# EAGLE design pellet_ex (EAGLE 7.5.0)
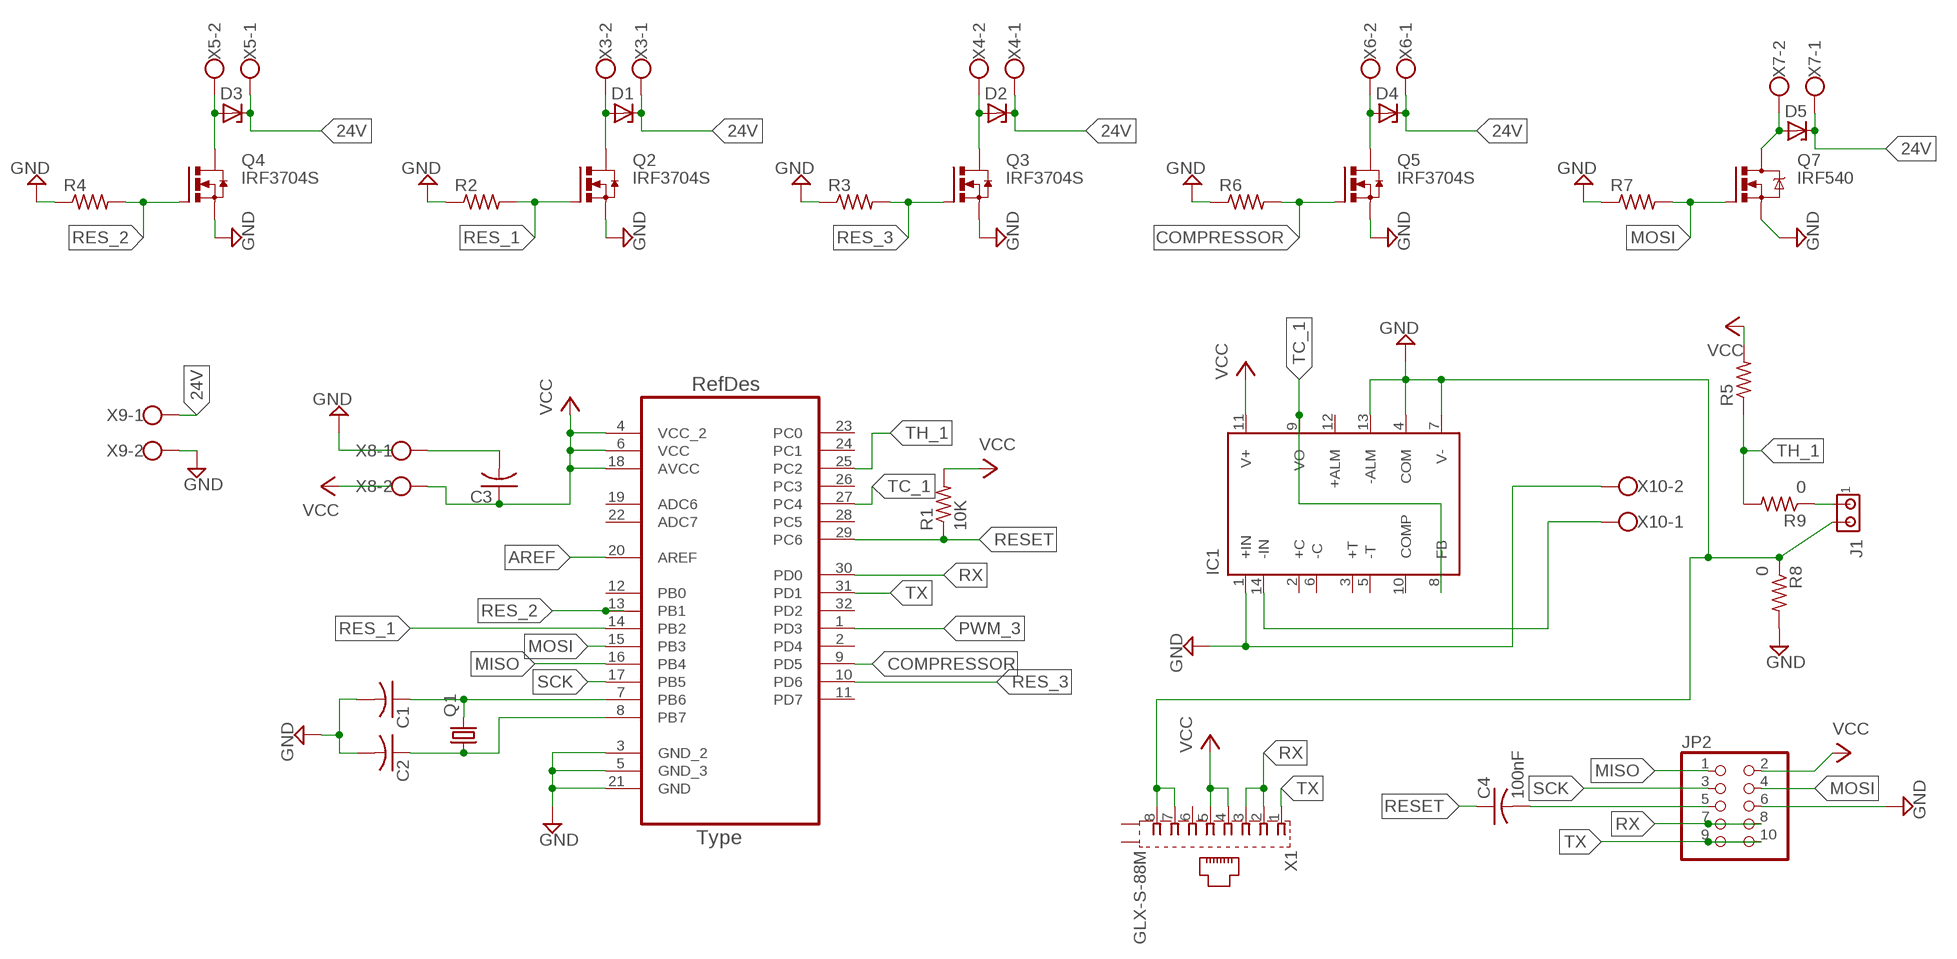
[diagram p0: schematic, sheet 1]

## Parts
C1  C-USC1206K  [C1206K]
C2  C-USC1206K  [C1206K]
C3  C-USC1206K  [C1206K]
C4  100nF  C-USC1206  [C1206]
D1  ZENER_DIODESOD123  [SOD123]
D2  ZENER_DIODESOD123  [SOD123]
D3  ZENER_DIODESOD123  [SOD123]
D4  ZENER_DIODESOD123  [SOD123]
D5  ZENER_DIODESOD123  [SOD123]
IC1  AD594  [DIL14]
J1  MTA02-156  [1X2MTA]
JP2  PINHD-2X5SMT  [2X05_SMT]
Q1  CRYSTALSM49  [SM49]
Q2  IRF3704S  [D2PACK]
Q3  IRF3704S  [D2PACK]
Q4  IRF3704S  [D2PACK]
Q5  IRF3704S  [D2PACK]
Q7  IRF540  [TO220BV]
R1  10K  R-US_M1206  [M1206]
R2  R-US_M1206  [M1206]
R3  R-US_M1206  [M1206]
R4  R-US_M1206  [M1206]
R5  R-US_M1206  [M1206]
R6  R-US_M1206  [M1206]
R7  R-US_M1206  [M1206]
R8  0  R-US_M1206  [M1206]
R9  0  R-US_M1206  [M1206]
U1  ATMEGA328P-AU  [QFP80P900X900X120-32N]
X1  GLX-S-88M  [GLX-S-88M]
X3  W237-102  [W237-102]
X4  W237-102  [W237-102]
X5  W237-102  [W237-102]
X6  W237-102  [W237-102]
X7  W237-102  [W237-102]
X8  W237-102  [W237-102]
X9  W237-102  [W237-102]
X10  W237-102  [W237-102]

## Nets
24V: D1.CATHODE D2.CATHODE D3.CATHODE D4.CATHODE D5.CATHODE X3.1 X4.1 X5.1 X6.1 X7.1 X9.1
AREF: U1.20(AREF)
COMPRESSOR: Q5.1(G) R6.2 U1.9(PD5)
GND: C1.2 C2.2 IC1.1(+IN) IC1.4(COM) IC1.7(V-) IC1.13(-ALM) J1.2 JP2.6 Q2.3(S) Q3.3(S) Q4.3(S) Q5.3(S) Q7.S R2.1 R3.1 R4.1 R6.1 R7.1 R8.1 R8.2 U1.3(GND_2) U1.5(GND_3) U1.21(GND) X1.7 X1.8 X9.2 X10.2
MISO: JP2.1 U1.16(PB4)
MOSI: JP2.4 Q7.G R7.2 U1.15(PB3)
N$1: IC1.14(-IN) X10.1
N$2: C1.1 Q1.2 U1.7(PB6)
N$3: C2.1 Q1.1 U1.8(PB7)
N$4: D1.ANODE Q2.2(D) X3.2
N$5: D2.ANODE Q3.2(D) X4.2
N$6: D3.ANODE Q4.2(D) X5.2
N$7: C4.2 JP2.5
N$8: D4.ANODE Q5.2(D) X6.2
N$9: D5.ANODE Q7.D X7.2
N$10: C3.2 X8.1
N$13: J1.1 R9.1
PWM_3: U1.1(PD3)
RES_1: Q2.1(G) R2.2 U1.14(PB2)
RES_2: Q4.1(G) R4.2 U1.13(PB1)
RES_3: Q3.1(G) R3.2 U1.10(PD6)
RESET: C4.1 R1.1 U1.29(PC6)
RX: JP2.7 JP2.8 U1.30(PD0) X1.2 X1.3
SCK: JP2.3 U1.17(PB5)
TC_1: IC1.8(FB) IC1.9(VO) U1.27(PC4)
TH_1: R5.1 R9.2 U1.25(PC2)
TX: JP2.9 JP2.10 U1.31(PD1) X1.1
VCC: C3.1 IC1.11(V+) JP2.2 R1.2 R5.2 U1.4(VCC_2) U1.6(VCC) U1.18(AVCC) X1.4 X1.5 X8.2
Unconnected: IC1.2(+C) IC1.3(+T) IC1.5(-T) IC1.6(-C) IC1.10(COMP) IC1.12(+ALM) U1.2(PD4) U1.11(PD7) U1.12(PB0) U1.19(ADC6) U1.22(ADC7) U1.23(PC0) U1.24(PC1) U1.26(PC3) U1.28(PC5) U1.32(PD2) X1.6 X1.S1 X1.S2

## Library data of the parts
C1-C4 = adafruit:C-US: CAPACITOR, American symbol
D1-D5 = fab:ZENER_DIODE: zener diode
IC1 = analog-devices:AD594: ANALOG DEVICES; MF: ALTERA CORPORATION; MPN: AD594AQ; OC_FARNELL: 409182; OC_NEWARK: 05F7088
J1 = con-amp:MTA02-156: AMP connector
JP2 = pinhead+:PINHD-2X5: PIN HEADER
Q1 = adafruit:CRYSTAL: CRYSTAL; OC_FARNELL: unknown; OC_NEWARK: unknown
Q2-Q5 = transistor-power:IRF3704: SMPS MOSFET HEXFET® Power MOSFET Source: http://www.irf.com/product-info/datasheets/data/irf3704.pdf
Q7 = transistor-power:IRF540: HEXFET Power MOSFET
R1-R9 = adafruit:R-US_: RESISTOR, American symbol
U1 = ATMEGA328P-AU:ATMEGA328P-AU; DESCRIPTION: 8-bit Microcontroller with In-System Programmable Flash; MPN: ATMEGA328P-AU; OC_FARNELL: 1715486; OC_NEWARK: 14R4631; PACKAGE: TQFP-32; SUPPLIER: Atmel
X1 = con-kycon:GLX-S-88M: Mod. Jack, Right Angle, 8 posiotion, 8 contatcs RJ45 Source: GLX-S-88M.pdf; OC_FARNELL: unknown; OC_NEWARK: unknown
X3-X10 = con-wago-500:W237-102: WAGO SCREW CLAMP; MPN: 237-102; OC_FARNELL: unknown; OC_NEWARK: 70K9898

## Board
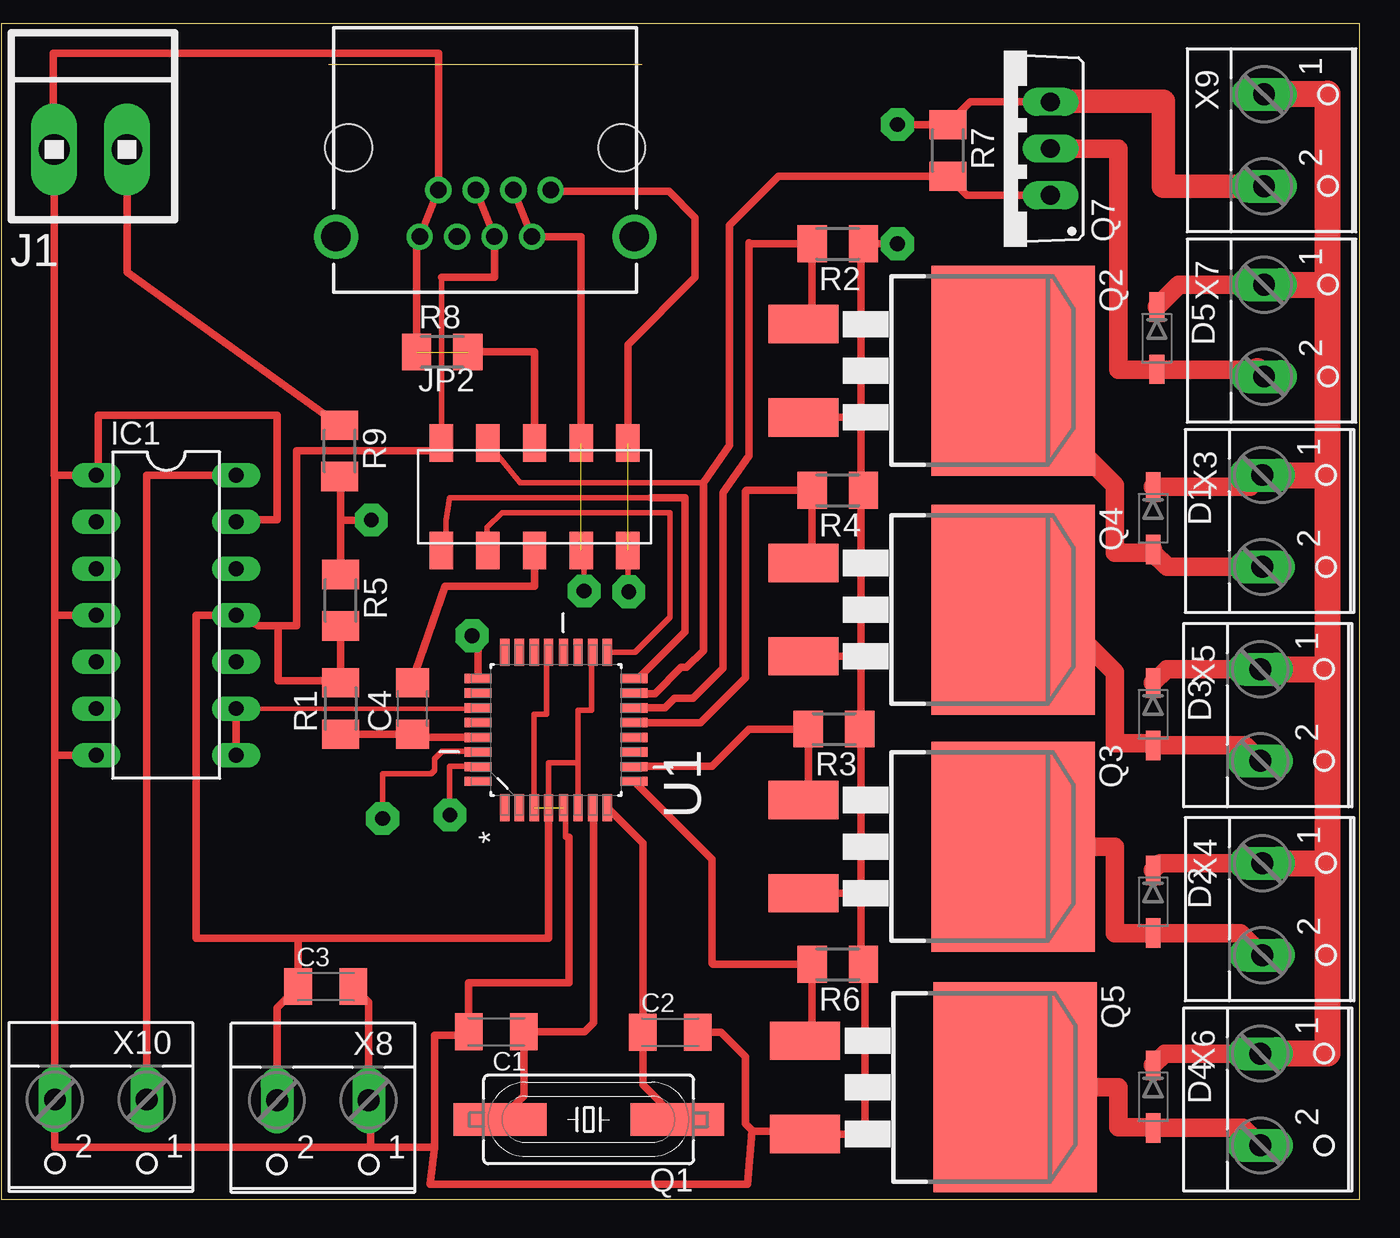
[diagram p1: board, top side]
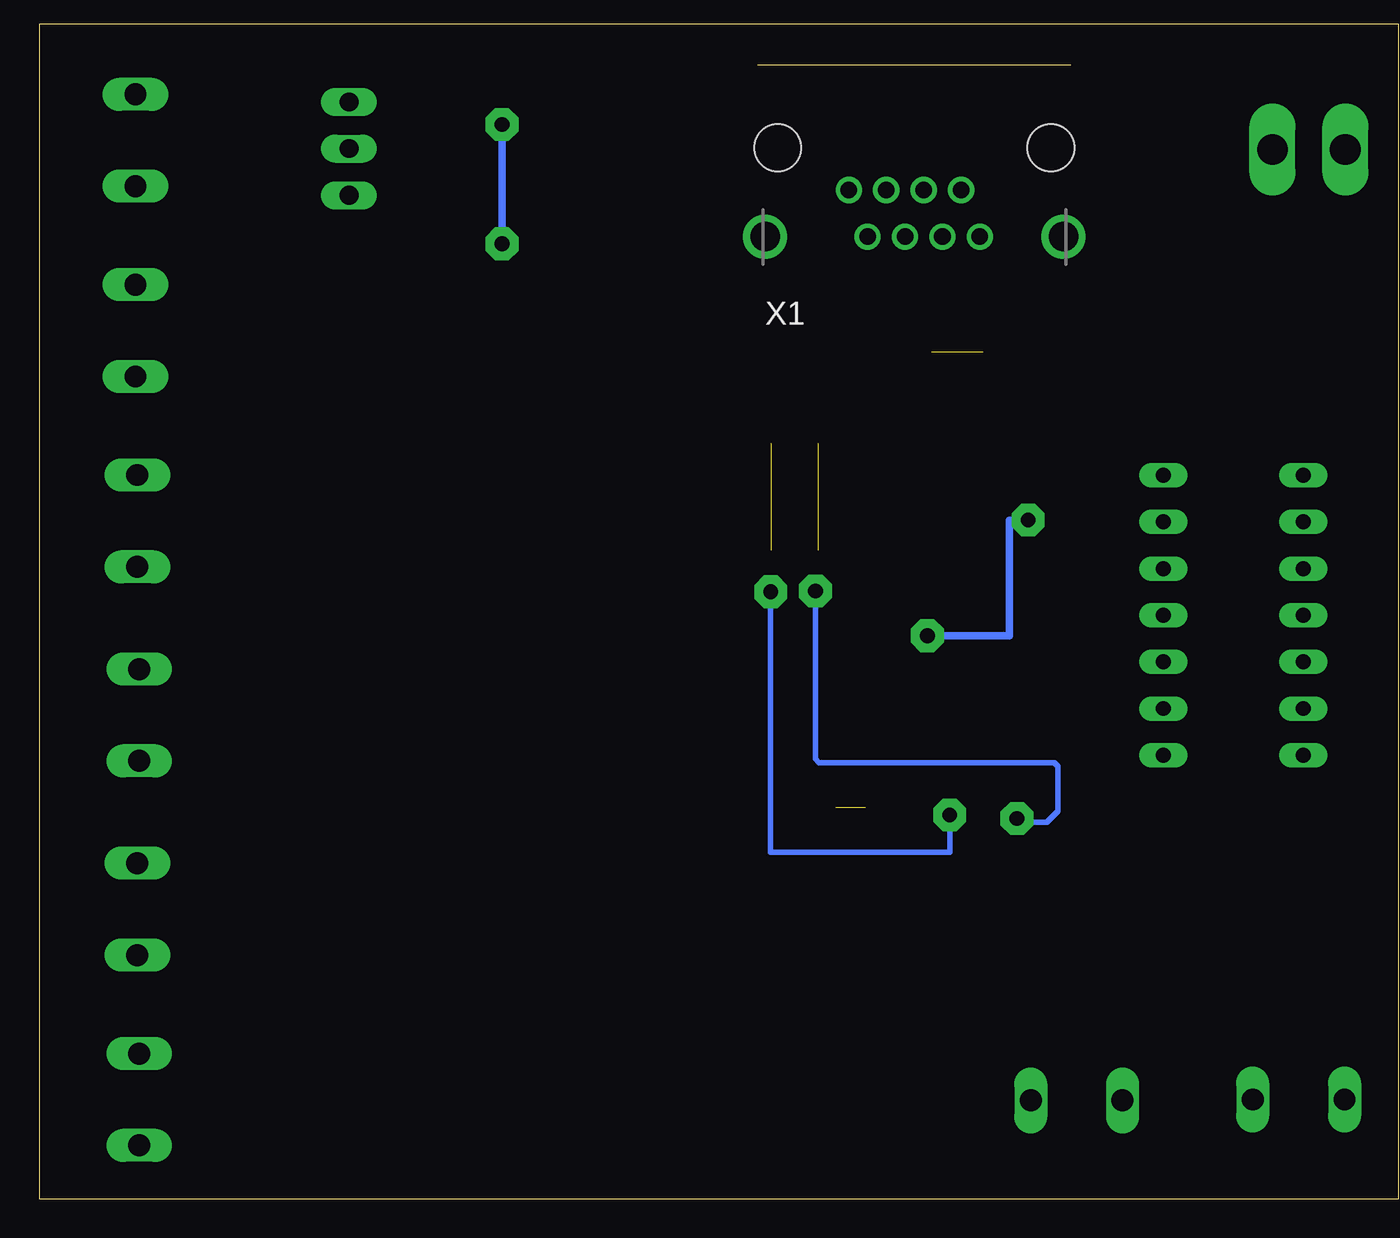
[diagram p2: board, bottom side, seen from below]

Size 17.06 x 0 mm. Coordinates in mm from the lower left corner, seen from the top.
Copper layers (1*16): Top 0.035mm / dielectric 1.5mm / Bottom 0.035mm
Design rules "default": minimum track width 10mil, minimum drill 24mil, track to track 8mil, track to pad 8mil, pad to pad 8mil, via to via 8mil, smd to smd 8mil, copper to edge 40mil, drill to drill 8mil, minimum pad ring 10mil, minimum via ring 8mil, stop-mask expansion 4mil, vias tented up to drill 0mil, thermal gap 10mil
Milling: 4 lines

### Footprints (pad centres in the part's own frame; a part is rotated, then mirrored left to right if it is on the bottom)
C1206K = smd 1.5 x 2: 1 -1.5,0; 2 1.5,0
C1206 = smd 1.6 x 1.8: 1 -1.4,0; 2 1.4,0
SOD123 = smd 1.6 x 0.8: ANODE 1.7,0; CATHODE -1.7,0
DIL14 = drill 0.813 long: 1 -7.62,-3.81; 2 -5.08,-3.81; 3 -2.54,-3.81; 4 0,-3.81; 5 2.54,-3.81; 6 5.08,-3.81; 7 7.62,-3.81; 8 7.62,3.81; 9 5.08,3.81; 10 2.54,3.81; 11 0,3.81; 12 -2.54,3.81; 13 -5.08,3.81; 14 -7.62,3.81
1X2MTA = drill 1.676 long: 1 1.981,0; 2 -1.981,0
2X05_SMT = smd 1.27 x 2.032: 1 -5.08,-2.921; 2 -5.08,2.921; 3 -2.54,-2.921; 4 -2.54,2.921; 5 0,-2.921; 6 0,2.921; 7 2.54,-2.921; 8 2.54,2.921; 9 5.08,-2.921; 10 5.08,2.921
SM49 = smd 5.08 x 1.778: 1 -4.826,0; 2 4.826,0
D2PACK = smd 2.083 x 3.81: 1 -2.54,-8.89; 3 2.54,-8.89 | smd 11.43 x 8.89: 2 0,2.54
TO220BV = drill 1.016 long: D 0,-2.54; G -2.54,-2.54; S 2.54,-2.54
M1206 = smd 1.6 x 2: 1 -1.4,0; 2 1.4,0
QFP80P900X900X120-32N = smd 1.473 x 0.508: 1 -4.242,2.794; 2 -4.242,2.007; 3 -4.242,1.194; 4 -4.242,0.406; 5 -4.242,-0.406; 6 -4.242,-1.194; 7 -4.242,-2.007; 8 -4.242,-2.794; 17 4.242,-2.794; 18 4.242,-2.007; 19 4.242,-1.194; 20 4.242,-0.406; 21 4.242,0.406; 22 4.242,1.194; 23 4.242,2.007; 24 4.242,2.794 | smd 0.508 x 1.473: 9 -2.794,-4.242; 10 -2.007,-4.242; 11 -1.194,-4.242; 12 -0.406,-4.242; 13 0.406,-4.242; 14 1.194,-4.242; 15 2.007,-4.242; 16 2.794,-4.242; 25 2.794,4.242; 26 2.007,4.242; 27 1.194,4.242; 28 0.406,4.242; 29 -0.406,4.242; 30 -1.194,4.242; 31 -2.007,4.242; 32 -2.794,4.242
GLX-S-88M = drill 0.9 pad 1.422: 1 -3.57,-2.3; 2 -2.55,-4.84; 3 -1.53,-2.3; 4 -0.51,-4.84; 5 0.51,-2.3; 6 1.53,-4.84; 7 2.55,-2.3; 8 3.57,-4.84 | drill 1.6 pad 2.184: S1 -8.125,-4.84; S2 8.125,-4.84 | hole 2.55: -7.44,0; 7.44,0
W237-102 = drill 1.194 long: 1 -2.5,-1.27; 2 2.5,-1.27

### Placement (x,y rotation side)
C1  9.14,-52.65 180 top  (outside the outline)
C2  18.62,-52.68 0 top  (outside the outline)
C3  -0.15,-50.19 0 top  (outside the outline)
C4  4.57,-35.05 90 top  (outside the outline)
D1  44.9,-24.69 270 top  (outside the outline)
D2  44.9,-45.57 270 top  (outside the outline)
D3  44.9,-35.36 270 top  (outside the outline)
D4  44.9,-56.18 270 top  (outside the outline)
D5  45.11,-14.88 270 top  (outside the outline)
IC1  -8.84,-29.97 270 top  (outside the outline)
J1  -12.96,-4.62 0 top  (outside the outline)
JP2  11.22,-23.52 0 top  (outside the outline)
Q1  14.17,-57.43 180 top  (outside the outline)
Q2  34.74,-16.66 270 top  (outside the outline)
Q3  34.74,-42.57 270 top  (outside the outline)
Q4  34.74,-29.67 270 top  (outside the outline)
Q5  34.85,-55.68 270 top  (outside the outline)
Q7  36.78,-4.57 90 top  (outside the outline)
R1  0.66,-35.05 90 top  (outside the outline)
R2  27.73,-9.75 180 top  (outside the outline)
R3  27.53,-36.17 180 top  (outside the outline)
R4  27.73,-23.16 180 top  (outside the outline)
R5  0.66,-29.16 270 top  (outside the outline)
R6  27.73,-48.97 180 top  (outside the outline)
R7  33.73,-4.67 270 top  (outside the outline)
R8  6.2,-15.65 0 top  (outside the outline)
R9  0.61,-21.03 270 top  (outside the outline)
U1  12.39,-36.22 90 top  (outside the outline)
X1  8.53,-4.52 0 bottom  (outside the outline)
X3  52.12,-24.84 270 top  (outside the outline)
X4  52.12,-45.97 270 top  (outside the outline)
X5  52.02,-35.41 270 top  (outside the outline)
X6  52.02,-56.34 270 top  (outside the outline)
X7  52.22,-14.48 270 top  (outside the outline)
X8  -0.31,-57.66 180 top  (outside the outline)
X9  52.22,-4.11 270 top  (outside the outline)
X10  -12.4,-57.61 180 top  (outside the outline)

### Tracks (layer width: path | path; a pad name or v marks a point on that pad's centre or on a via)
24V
  Top 1.016: D5.CATHODE 46.31,-11.98 X7.1 | X3.1 50.2,-22.99 D1.CATHODE | X5.1 45.65,-32.91 D3.CATHODE | X4.1 45.3,-43.47 D2.CATHODE | X6.1 45.55,-53.84 D4.CATHODE
  Top 1.422: X9.1 50.95,-1.57 54.4,-1.57 54.4,-11.98 | 54.4,-11.98 54.4,-22.34 | 54.4,-22.34 54.4,-32.91 | 54.4,-32.91 54.4,-43.47 | 54.4,-43.47 54.4,-53.84 X6.1 | X4.1 54.4,-43.47 | X5.1 54.4,-32.91 | X3.1 54.4,-22.34 | X7.1 54.4,-11.98
COMPRESSOR
  Top 0.406: U1.9 20.88,-43.25 20.88,-48.92 20.93,-48.97 R6.2 26.33,-52.76 Q5.1
GND  (via drill 0.8 pad 1.78)  (2 unrouted)
  Top 0.305: 13.1,-42.06 12.9,-42.06 12.9,-40.46 U1.5 | U1.3 11.2,-35.36 11.88,-35.36 11.88,-31.98 U1.21
  Top 0.406: Q7.S 34.97,-2.03 R7.1 30.99,-3.27 v30.99,-3.25 | 29,-19.25 29,-9.88 R2.1 v30.99,-9.75 | 29,-19.25 28.95,-19.2 Q2.3 | 29,-19.25 29,-23.03 R4.1 29,-23.29 29,-32.26 | 29,-32.26 28.95,-32.21 Q4.3 | 29,-32.26 29,-36.1 R3.1 29,-36.24 29,-45.06 | 29,-45.06 28.95,-45.11 Q3.3 | 29,-45.06 29,-48.84 R6.1 29.21,-49.04 29.21,-58.27 29.16,-58.22 Q5.3 25.96,-58.06 23.11,-58.06 | 20.12,-52.81 C2.2 21.38,-52.68 22.7,-54 22.7,-57.66 23.11,-58.06 | 5.79,-58.93 5.79,-52.83 7.64,-52.83 C1.2 7.64,-49.99 13.1,-49.99 13.1,-42.06 | 5.79,-58.93 5.54,-60.95 22.81,-60.95 23.06,-58.06 23.11,-58.06 | 2.28,-56.29 2.28,-58.93 | 2.28,-58.93 5.79,-58.93 | 2.28,-58.93 -14.9,-58.93 X10.2 -14.9,-37.59 | JP2.6 11.23,-15.64 R8.2 | IC1.1 -14.9,-22.35 -14.9,-29.97 | -14.9,-29.97 -14.9,-37.59 | IC1.7 -14.9,-37.59 | IC1.4 -14.9,-29.97 | IC1.1 -12.55,-22.35 -12.55,-19.1 -2.79,-19.1 -2.79,-19.3 -2.79,-24.79 -5.03,-24.79 IC1.13 | R8.1 4.79,-9.36 X1.8 X1.7 5.98,0.61 -14.98,0.61 -14.98,-4.62 J1.2 -14.94,-22.35 IC1.1
  Top 1.27: X9.2 45.46,-6.61 45.46,-1.98 39.32,-1.98 Q7.S
  Bottom 0.406: v30.99,-9.75 v30.99,-3.25
MISO
  Top 0.305: 17.57,-23.57 6.6,-23.57 6.4,-24.79 6.4,-26.19 JP2.1
  Top 0.406: U1.16 16.86,-33.43 19.4,-30.89 19.4,-23.57 17.57,-23.57
MOSI
  Top 0.305: 20.42,-22.76 10.44,-22.76 JP2.4
  Top 0.406: Q7.G 34.77,-7.11 R7.2 24.51,-6.07 21.84,-8.74 21.84,-20.73 20.42,-22.76 20.42,-31.9 19.5,-32.82 19.2,-32.82 17.78,-34.24 16.63,-34.24 U1.15
N$1
  Top 0.406: X10.1 -9.9,-41.45 -9.9,-22.35 IC1.14
N$2
  Top 0.406: Q1.2 10.64,-56.13 C1.1 13.94,-52.65 14.42,-52.17 14.42,-40.49 U1.7
N$3
  Top 0.406: Q1.1 17.12,-55.55 C2.1 17.12,-42.39 U1.8
N$4
  Top 1.016: Q2.2 37.28,-17.37 42.82,-22.91 42.82,-26.57 44.9,-26.57 | 44.9,-26.57 D1.ANODE | 44.9,-26.57 45.68,-27.34 X3.2
N$5
  Top 1.016: Q3.2 42.82,-42.57 42.82,-47.29 44.9,-47.29 | 44.9,-47.29 D2.ANODE | 44.9,-47.29 49.67,-47.29 X4.2
N$6
  Top 1.016: X5.2 49.9,-37.06 D3.ANODE 44.9,-36.93 42.82,-36.93 42.82,-33.07 39.42,-29.67 Q4.2
N$7
  Top 0.406: JP2.5 11.22,-28.4 6.35,-28.4 4.52,-33.65 C4.2
N$8
  Top 1.016: X6.2 49.79,-57.88 D4.ANODE 44.9,-57.86 43.02,-57.86 43.02,-55.68 Q5.2
N$9
  Top 1.016: Q7.D 43.02,-4.57 43.02,-16.61 45.11,-16.61 50.58,-16.61
  Top 1.27: 45.11,-16.61 D5.ANODE | 50.58,-16.61 X7.2
N$10
  Top 0.406: X8.1 2.19,-51.04 C3.2
N$13
  Top 0.406: J1.1 -10.98,-11.3 R9.1
RES_1
  Top 0.406: Q2.1 26.33,-13.64 R2.2 22.96,-9.75 22.91,-9.7 22.91,-21.28 21.49,-23.32 21.49,-32.87 19.86,-34.49 18.84,-34.49 18.34,-35 16.66,-35 U1.14
RES_2
  Top 0.406: Q4.1 26.33,-26.65 R4.2 22.76,-23.16 22.7,-23.21 22.7,-33.37 20.27,-35.81 U1.13
RES_3
  Top 0.406: Q3.1 26.13,-39.75 R3.2 22.91,-36.17 20.88,-38.2 16.71,-38.2 16.66,-38.25 U1.10
RESET
  Top 0.406: U1.29 4.74,-36.63 C4.1 R1.1
RX  (via drill 0.8 pad 1.78)  (1 unrouted)
  Top 0.305: U1.30 8.13,-37.39 6.19,-37.39 5.79,-37.79 5.79,-38.4 5.59,-38.61 2.94,-38.61 v2.94,-41.05 | v13.92,-28.65 13.92,-26.44 JP2.7
  Top 0.406: X1.3 X1.2 13.76,-9.36 JP2.8
  Bottom 0.305: v2.94,-41.05 2.74,-41.25 1.32,-41.25 0.71,-40.64 0.71,-38.2 0.91,-38 13.71,-38 13.92,-37.79 v13.92,-28.65
SCK
  Top 0.305: U1.17 16.69,-31.98 18.59,-30.07 18.59,-24.38 9.45,-24.38 8.63,-25.2 8.63,-26.39 JP2.3
TC_1
  Top 0.254: 8.15,-35.05 IC1.9
  Top 0.406: U1.27 8.15,-35.05 | IC1.9 IC1.8
TH_1  (via drill 0.8 pad 1.78)
  Top 0.406: U1.25 8.15,-31.09 v7.82,-31.09 | R5.1 0.66,-24.79 | 0.66,-24.79 0.66,-22.43 R9.2 | v2.33,-24.79 0.66,-24.79
  Bottom 0.406: v7.82,-31.09 3.35,-31.09 3.35,-24.79 v2.33,-24.79
TX  (via drill 0.8 pad 1.78)  (1 unrouted)
  Top 0.305: U1.31 8.15,-38.2 6.6,-38.2 v6.6,-40.84 | JP2.9 16.3,-28.4 v16.35,-28.7
  Top 0.406: JP2.10 16.3,-15.24 19.97,-11.58 19.97,-8.33 18.54,-6.9 12.19,-6.9 X1.1
  Bottom 0.305: v6.6,-40.84 6.6,-42.87 16.35,-42.87 v16.35,-28.7
VCC
  Top 0.305: U1.6 13.59,-38 | 13.59,-38 13.59,-35.15 14.32,-35.15 14.32,-31.98 U1.18 | U1.4 11.99,-38 13.59,-38 | JP2.2 6.15,-11.58
  Top 0.406: X8.2 -2.81,-51.34 C3.1 -1.66,-47.55 | -1.66,-47.55 11.99,-47.55 U1.4 | -1.66,-47.55 -7.22,-47.55 -7.22,-29.97 IC1.11 -3.84,-30.56 -2.75,-30.56 | -2.75,-30.56 -1.73,-30.56 -1.73,-21.03 6.14,-21.03 JP2.2 | R1.2 0.66,-33.53 | 0.66,-33.53 -2.75,-33.53 -2.75,-30.56 | 0.66,-33.53 R5.2 | 6.15,-11.58 9.04,-11.58 X1.4 X1.5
